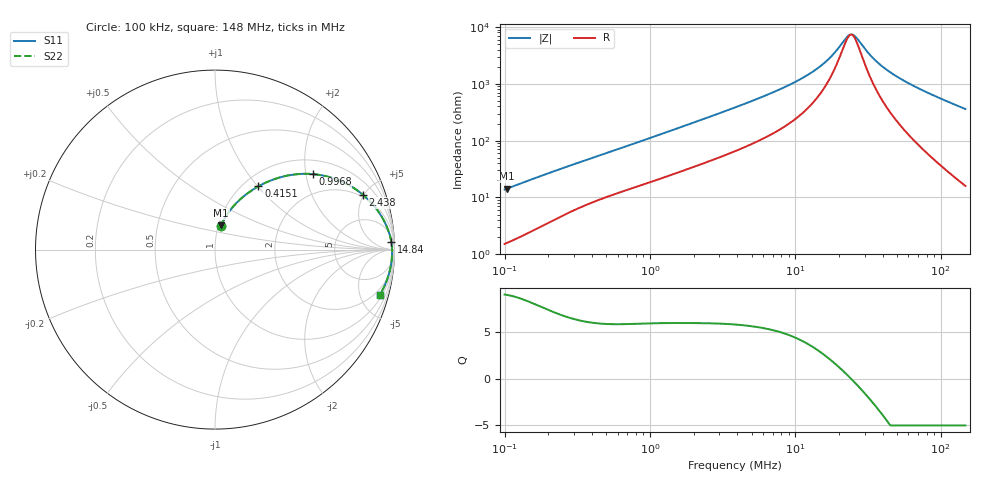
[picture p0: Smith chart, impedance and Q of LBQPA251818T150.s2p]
! LBQPA251818T150  S-PARAMETER MODEL  ( General Type )
! Model Generated by TAIYO YUDEN Corporation (http://www.ty-top.com)
! Version 1.0
! TAIYO YUDEN Control No. 191025NI43SB-FBB
! Copyright(c) 2019 TAIYO YUDEN CO.,LTD. All Rights Reserved.
! Product Description (link to TY-COMPAS)
! https://ds.yuden.co.jp/TYCOMPAS/or/detail?pn=LBQPA251818T150K&u=M
! Products Name : Inductors
! Characteristics :
!  Inductance : 15 uH , SRF(min) : 23 MHz , DC Resistance(max) : 0.845 Ohm
!  Rated Current : Saturation :350 mA , Temp Rise : 285 mA (20 degC)
!  Case Size : 2.5 x 1.8 / 0.098 x 0.071 [mm/inch] , Thickness : 1.8 / 0.071 [mm/inch]
!  (Conditions: Temperature = 25 degC , DC Bias Current/Voltage = 0A / 0V)
! External Node Assignments :
!  1  o---GGG---o  2
! GND o---------o GND
! Frequency Range : 0.1MHz  -  147.97148MHz  [ 402 STEP ]
# MHz S RI R 50
! Freq[MHz].  S11 Real  S11 Imag  S21 Real  S21 Imag  S12 Real  S12 Imag  S22 Real  S22 Imag
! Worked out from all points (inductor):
!   401 points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, 100 kHz to 148 MHz, reference 50 ohm
!   read as one part in series: L = 21.6 uH near 103.7 kHz
!   highest Q = 8.96 at 103.7 kHz (marker M1), where L = 21.8 uH
!   self-resonance near 24.19 MHz
!   S11 on the Smith chart (normalised r, x): 100 kHz: 1.03, +0.27; 415.1 kHz: 1.17, +1.01; 996.8 kHz: 1.37, +2.19; 2.438 MHz: 1.83, +4.92; 14.84 MHz: 14, +38; 148 MHz: 1.32, -7.19
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0.1  0.0327 0.1307  0.9673 -0.1307  0.9673 -0.1307  0.0327 0.1307
0.103717  0.0345 0.1351  0.9655 -0.1351  0.9655 -0.1351  0.0345 0.1351
0.192893  0.0888 0.2252  0.9112 -0.2252  0.9112 -0.2252  0.0888 0.2252
0.339629  0.1914 0.3207  0.8086 -0.3207  0.8086 -0.3207  0.1914 0.3207
0.415131  0.2422 0.3526  0.7578 -0.3526  0.7578 -0.3526  0.2422 0.3526
0.667185  0.3928 0.4102  0.6072 -0.4102  0.6072 -0.4102  0.3928 0.4102
0.996796  0.5439 0.4207  0.4561 -0.4207  0.4561 -0.4207  0.5439 0.4207
1.153479  0.5989 0.4131  0.4011 -0.4131  0.4011 -0.4131  0.5989 0.4131
1.69217  0.7292 0.3683  0.2708 -0.3683  0.2708 -0.3683  0.7292 0.3683
2.437546  0.8244 0.3054  0.1756 -0.3054  0.1756 -0.3054  0.8244 0.3054
3.917549  0.9051 0.2192  0.0949 -0.2192  0.0949 -0.2192  0.9051 0.2192
7.98191  0.9631 0.1128  0.0369 -0.1128  0.0369 -0.1128  0.9631 0.1128
13.06453  0.9795 0.0576  0.0205 -0.0576  0.0205 -0.0576  0.9795 0.0576
14.84472  0.982 0.0449  0.018 -0.0449  0.018 -0.0449  0.982 0.0449
18.14478  0.9847 0.026  0.0153 -0.026  0.0153 -0.026  0.9847 0.026
22.58693  0.9863 0.00617  0.0137 -0.00617  0.0137 -0.00617  0.9863 0.00617
24.29735  0.9866 -0.000409  0.0134 0.000409  0.0134 0.000409  0.9866 -0.000409
26.1373  0.9868 -0.007  0.0132 0.007  0.0132 0.007  0.9868 -0.007
34.99999  0.9863 -0.0342  0.0137 0.0342  0.0137 0.0342  0.9863 -0.0342
44.37094  0.9843 -0.0583  0.0157 0.0583  0.0157 0.0583  0.9843 -0.0583
72.62492  0.9734 -0.1197  0.0266 0.1197  0.0266 0.1197  0.9734 -0.1197
147.9715  0.9187 -0.252  0.0813 0.252  0.0813 0.252  0.9187 -0.252
